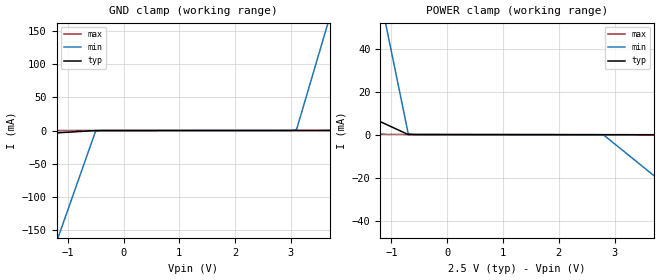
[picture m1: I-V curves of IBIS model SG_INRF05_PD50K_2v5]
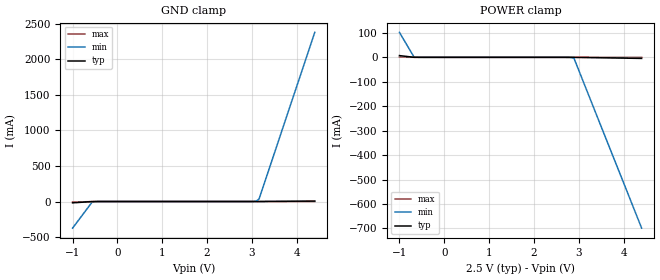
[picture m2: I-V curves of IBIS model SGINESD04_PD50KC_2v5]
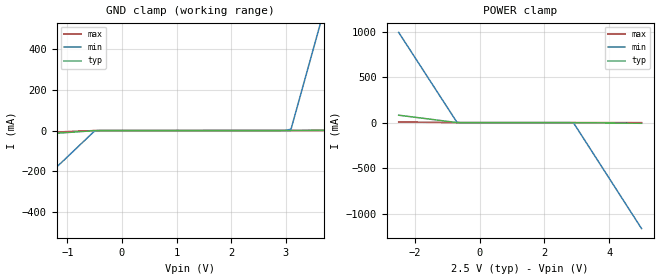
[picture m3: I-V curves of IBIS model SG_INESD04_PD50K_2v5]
|   This file is an IBIS representation of the   |
|   Integrated Device Technology, Inc.   |
|   ICS850S1201I   |
|   12:1 SINGLE-ENDED MULTIPLEXER   |
[IBIS Ver]   4.1
[File name]   850s1201i.ibs
[File Rev]   1.0
[Date]   14 Jan 2010
[Source]   Originated at Integrated Device Technology, Inc.
[Disclaimer]
IDT hereby grants the user of this IBIS model a non-exclusive,
nontransferable license to use this IBIS model under the following terms.
Before using this IBIS model, the user should read this license.
If the user does not accept these terms,  the IBIS model should be
returned to IDT within 30 days.
   The user is granted this license only to use the IBIS model and
is not granted rights to sell, load, rent, lease or license the IBIS
model in whole or in part, or in modified form to anyone other than
user. User may modify the IBIS model to suit its specific
applications but rights to derivative works and such modifications
shall belong to IDT.
   This IBIS model is provided on an "AS IS" basis and IDT makes
absolutely no warranty with respect to the information contained
herein. IDT DISCLAIMS AND CUSTOMER WAIVES ALL WARRANTIES, EXPRESS
OR IMPLIED, INCLUDING WARRANTIES OF MERCHANTABILITY OR FITNESS FOR
A PARTICULAR PURPOSE. The entire risk as to quality and performance
is with the Customer. ACCORDINGLY, IN NO EVENT SHALL THE COMPANY BE
LIABLE FOR ANY DAMAGES, WHETHER IN CONTRACT OR TORT,INCLUDING ANY
LOST PROFITS OR OTHER INCIDENTAL, CONSEQUENTIAL, EXEMPLARY, OR
PUNITIVE DAMAGES ARISING OUT OF THE USE OR APPLICATION OF THE IBIS
model provided in this package. Further, IDT reserves the right to
make changes without notice to any product herein to improve
reliability, function, or design. IDT does not convey any license
under patent rights or any other intellectual property rights,
including those of third parties.
   IDT is not obligated to provide maintenance or support
for the licensed IBIS model.
[Copyright]   Copyright 2005 by Integrated Device Technology, Inc.
[Component]   ICS874001GI-05
[Manufacturer] Integrated Device Technology, Inc.
[Package]
|TSSOP 20 Lead
|   typ   min   max
R_pkg   51.85m   41.1m   62.6m
L_pkg   1.568nH   0.734nH   2.401nH
C_pkg   0.221pF   0.068pF   0.373pF
[Pin] signal_name   model_name   R_pin   L_pin   C_pin
1  CLK8   SG_INRF05_PD50K   62.6m   2.401n   0.373p
2  CLK9   SG_INRF05_PD50K   57.23m   1.985n   0.297p
3  CLK10   SG_INRF05_PD50K   51.85m   1.568n   0.221p
4  CLK11   SG_INRF05_PD50K   46.78m   1.151n   0.145p
5  VDD   POWER   41.1m   0.734n   0.068p
6  CLK_SEL0   SGINESD04_PD50KC   41.1m   0.734n   0.068p
7  CLK_SEL1   SGINESD04_PD50KC   46.78m   1.151n   0.145p
8  CLK_SEL2   SG_INESD04_PD50K   51.85m   1.568n   0.221p
9  CLK_SEL3   SG_INESD04_PD50K   57.23m   1.985n   0.297p
10 OE   SG_INESD04_PU50K   62.6m   2.401n   0.373p
11 Q   SG_COUT02_15OHM_   62.6m   2.401n   0.373p
12 GND   GND   57.23m   1.985n   0.297p
13 CLK0   SG_INRF05_PD50K   51.85m   1.568n   0.221p
14 CLK1   SG_INRF05_PD50K   46.78m   1.151n   0.145p
15 CLK2   SG_INRF05_PD50K   41.1m   0.734n   0.068p
16 CLK3   SG_INRF05_PD50K   41.1m   0.734n   0.068p
17 CLK4   SG_INRF05_PD50KC   46.78m   1.151n   0.145p
18 CLK5   SG_INRF05_PD50K   51.85m   1.568n   0.221p
19 CLK6   SG_INRF05_PD50K   57.23m   1.985n   0.297p
20 CLK7   SG_INRF05_PD50K   62.6m   2.401n   0.373p
[Model Selector] SG_INRF05_PD50K
SG_INRF05_PD50K_2v5  Buffer selection for 2v5
SG_INRF05_PD50K_3v3  Buffer selection for 3v3
[Model Selector] SGINESD04_PD50KC
SGINESD04_PD50KC_2v5  Buffer selection for 2v5
SGINESD04_PD50KC_3v3  Buffer selection for 3v3
[Model Selector] SG_INESD04_PD50K
SG_INESD04_PD50K_2v5  Buffer selection for 2v5
SG_INESD04_PD50K_3v3  Buffer selection for 3v3
[Model Selector] SG_INESD04_PU50K
SG_INESD04_PU50K_2v5  Buffer selection for 2v5
SG_INESD04_PU50K_3v3  Buffer selection for 3v3
[Model Selector] SG_COUT02_15OHM_
SG_COUT02_15OHM__2v5  Buffer selection for 2v5
SG_COUT02_15OHM__3v3  Buffer selection for 3v3
[Model Selector] SG_INRF05_PD50KC
SG_INRF05_PD50KC_2v5  Buffer selection for 2v5
SG_INRF05_PD50KC_3v3  Buffer selection for 3v3
| Models and submodels in the file (12): SG_INRF05_PD50K_2v5 (Input), SGINESD04_PD50KC_2v5 (Input), SG_INESD04_PD50K_2v5 (Input), SG_INESD04_PU50K_2v5 (Input), SG_COUT02_15OHM__2v5 (Output), SG_INRF05_PD50KC_2v5 (Input), SG_INRF05_PD50K_3v3 (Input), SGINESD04_PD50KC_3v3 (Input), SG_INESD04_PD50K_3v3 (Input), SG_INESD04_PU50K_3v3 (Input), SG_COUT02_15OHM__3v3 (Output), SG_INRF05_PD50KC_3v3 (Input)
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[Model] SG_INRF05_PD50K_2v5
Model_type   Input
Polarity   Non-Inverting
Vinl = 0.70V
Vinh = 1.7V
|   typ   min   max
C_comp   2pF   1.5pF   2.5pF
|   typ   min   max
[Voltage range]  2.5V   2.375V   2.625V
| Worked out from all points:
|   GND clamp passes 1 mA (typ) near -0.69 V on its own axis
|   POWER clamp passes 1 mA (typ) near -0.78 V on its own axis
[GND_clamp]
|Voltage   I(typ)   I(min)   I(max)
-2.5V     -10.13mA   -476.9mA   -65.78uA
-1.2V     -3.557mA   -167.5mA   -29.07uA
-1.1V     -3.052mA   -143.8mA   -26.25uA
-500mV    -20.42uA   -979.9uA   -9.306uA
3V        59.71uA    107.4uA    55.83uA
3.1V      62.2uA     1.223mA    57.7uA
3.6V      193.5uA    143.4mA    67.02uA
3.7V      219.7uA    171.8mA    68.88uA
5V        561.1uA    541.4mA    93.11uA
[POWER_clamp]
|Voltage   I(typ)   I(min)   I(max)
-2.5V     21.53mA    228.2mA    557.9uA
-1.1V     4.854mA    51.17mA    172.3uA
-1V       3.663mA    38.52mA    144.7uA
-700mV    88.46uA    578.9uA    62.07uA
-500mV    59.71uA    60.2uA     58.16uA
2.8V      -5.971uA   -94.12uA   -3.255uA
5V        -54.33uA   -46.22mA   -44.17uA
[Model] SGINESD04_PD50KC_2v5
Model_type   Input
Polarity   Non-Inverting
Vinl = 0.7V
Vinh = 1.7V
|   typ   min   max
C_comp   2pF   1.5pF   2.5pF
|   typ   min   max
[Voltage range]   2.5V   2.375V   2.625V
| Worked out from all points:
|   GND clamp passes 1 mA (typ) near -0.55 V on its own axis
|   POWER clamp passes 1 mA (typ) near -0.71 V on its own axis
[GND_clamp]
|Voltage   I (typ)   I (min)   I (max)
-999mV    -18.75mA   -374.8mA   -8.404mA
-564.6mV  -1.216mA   -9.414mA   -581.3uA
-502.5mV  -388.1uA   -1.754mA   -121.6uA
2.973V    59.47uA    274.3uA    55.12uA
3.097V    84.25uA    5.578mA    57.43uA
3.159V    162.4uA    35.91mA    58.66uA
4.4V      6.445mA    2.381A     98.18uA
[Power_clamp]
|Voltage   I (typ)   I (min)   I (max)
-999mV    7.129mA    102.1mA    575.6uA
-675.1mV  206.3uA    1.514mA    72.72uA
2.888V    -25.65uA   -2.311mA   -4.887uA
4.4V      -4.427mA   -698.7mA   -43.51uA
[Model] SG_INESD04_PD50K_2v5
Model_type   Input
Polarity   Non-Inverting
Vinl = 0.7V
Vinh = 1.7V
|   typ   min   max
C_comp   2pF   1.5pF   2.5pF
|   typ   min   max
[Voltage range]   2.5V   2.375V   2.625V
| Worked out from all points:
|   GND clamp passes 1 mA (typ) near -0.53 V on its own axis
|   POWER clamp passes 1 mA (typ) near -0.71 V on its own axis
[GND_clamp]
|Voltage   I (typ)   I (min)   I (max)
-2.5V     -37.48mA   -508.7mA   -20.53mA
-500mV    -417.5uA   -1.693mA   -161.7uA
2.9V      8.038uA    74.9uA     5.099uA
3.1V      53.32uA    6.625mA    8.822uA
3.6V      1.835mA    485.7mA    21.56uA
3.7V      2.191mA    581.5mA    24.11uA
5V        6.822mA    1.827A     57.22uA
[Power_clamp]
|Voltage   I (typ)   I (min)   I (max)
-2.5V     81.82mA    992.2mA    7.3mA
-700mV    409.6uA    3.352mA    52.39uA
2.9V      -83.01uA   -3.19mA    -53.78uA
5V        -7.106mA   -1.166A    -111.4uA
